(* Logix 5000 AddOnInstructionDefinition export Banner_S15C_UI_Param_v2; software revision 32.00; part 2 of 2 *)
(* tags used below, declared in another part *)
   S15C : Banner_S15C_UI_v2;
   Port_Data : Banner_IOL_Port_v2;
   Port : DINT;
   Local_Control : DINT;
   Command_Being_Processed : BOOL;
   Index_Write_Inprocess : INT;
   Update_Archive : BOOL;
   Inprocess_Index : DINT;
(* Banner_S15C_UI_Param_v2, continued *)

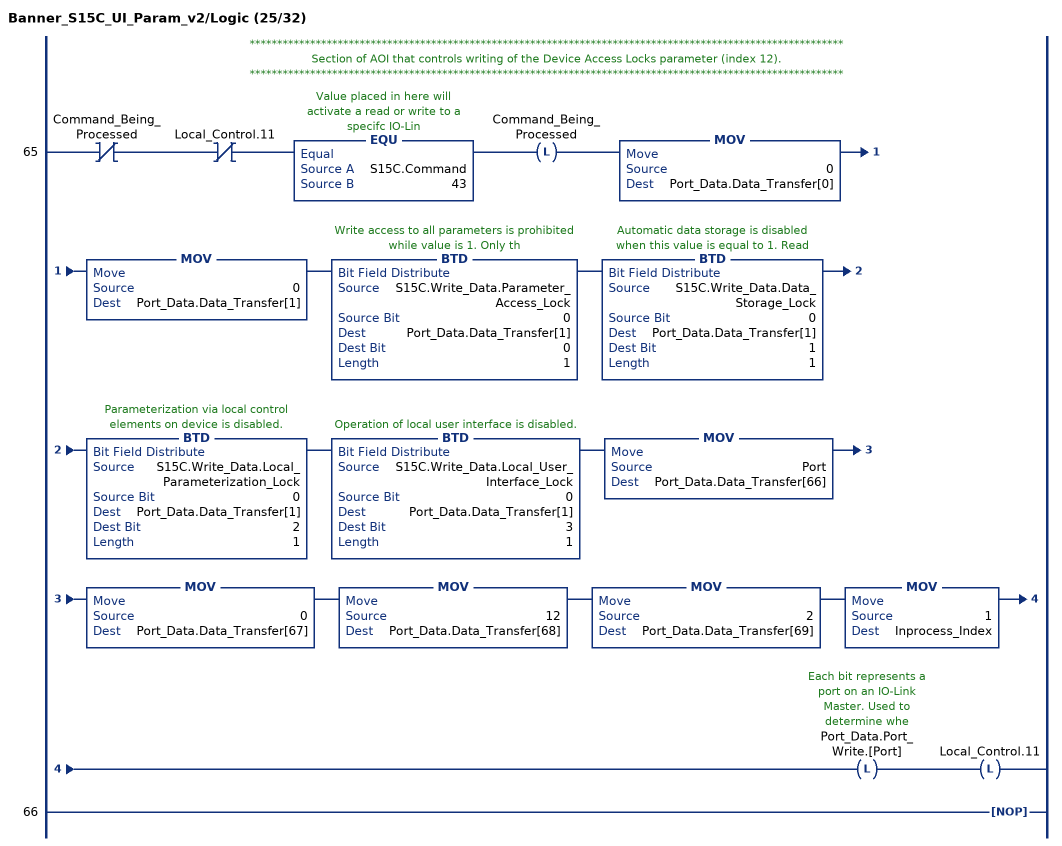
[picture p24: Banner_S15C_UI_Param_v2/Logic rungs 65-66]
   // ************************************************************************************************************
   // Section of AOI that controls writing of the Device Access Locks parameter (index 12).
   // ************************************************************************************************************
   65: XIO(Command_Being_Processed)XIO(Local_Control.11)EQU(S15C.Command,43)OTL(Command_Being_Processed)MOV(0,Port_Data.Data_Transfer[0])MOV(0,Port_Data.Data_Transfer[1])BTD(S15C.Write_Data.Parameter_Access_Lock,0,Port_Data.Data_Transfer[1],0,1)BTD(S15C.Write_Data.Data_Storage_Lock,0,Port_Data.Data_Transfer[1],1,1)BTD(S15C.Write_Data.Local_Parameterization_Lock,0,Port_Data.Data_Transfer[1],2,1)BTD(S15C.Write_Data.Local_User_Interface_Lock,0,Port_Data.Data_Transfer[1],3,1)MOV(Port,Port_Data.Data_Transfer[66])MOV(0,Port_Data.Data_Transfer[67])MOV(12,Port_Data.Data_Transfer[68])MOV(2,Port_Data.Data_Transfer[69])MOV(1,Inprocess_Index)OTL(Port_Data.Port_Write.[Port])OTL(Local_Control.11);
   66: NOP();
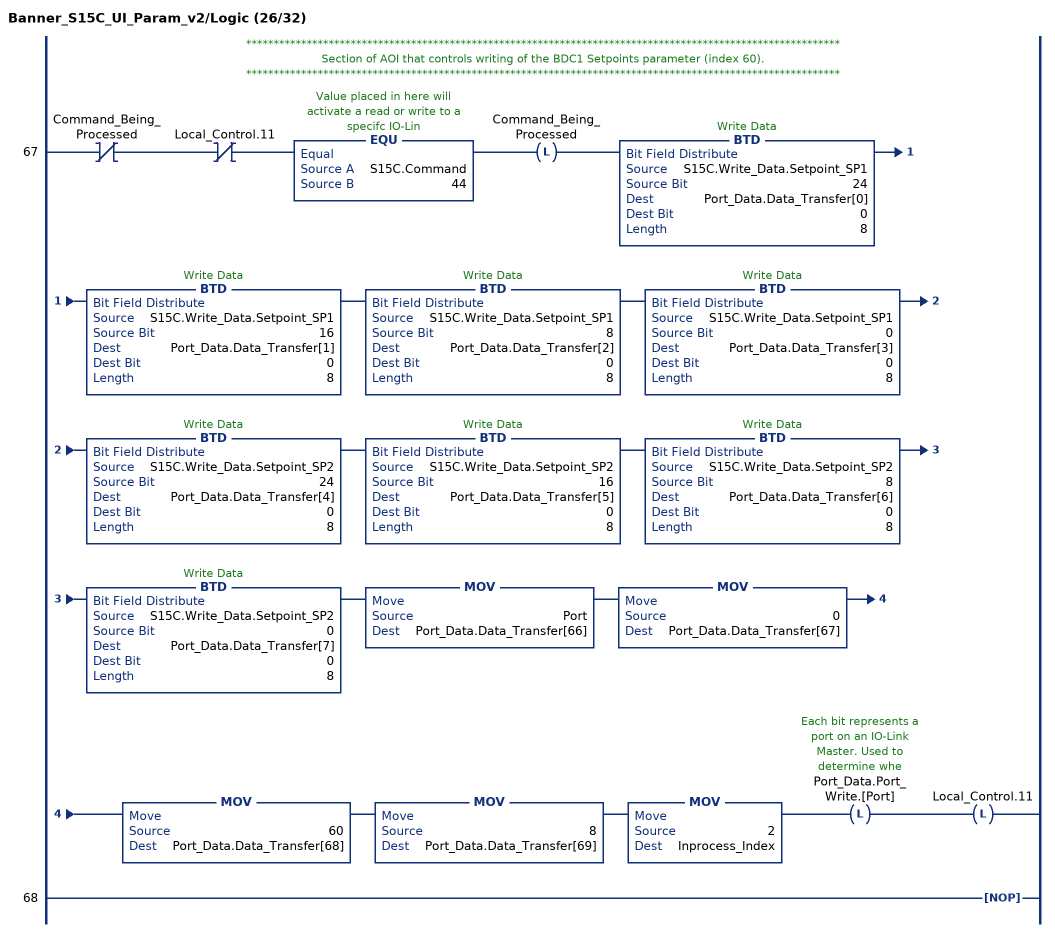
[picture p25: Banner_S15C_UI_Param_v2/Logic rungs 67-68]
   // ************************************************************************************************************
   // Section of AOI that controls writing of the BDC1 Setpoints parameter (index 60).
   // ************************************************************************************************************
   67: XIO(Command_Being_Processed)XIO(Local_Control.11)EQU(S15C.Command,44)OTL(Command_Being_Processed)BTD(S15C.Write_Data.Setpoint_SP1,24,Port_Data.Data_Transfer[0],0,8)BTD(S15C.Write_Data.Setpoint_SP1,16,Port_Data.Data_Transfer[1],0,8)BTD(S15C.Write_Data.Setpoint_SP1,8,Port_Data.Data_Transfer[2],0,8)BTD(S15C.Write_Data.Setpoint_SP1,0,Port_Data.Data_Transfer[3],0,8)BTD(S15C.Write_Data.Setpoint_SP2,24,Port_Data.Data_Transfer[4],0,8)BTD(S15C.Write_Data.Setpoint_SP2,16,Port_Data.Data_Transfer[5],0,8)BTD(S15C.Write_Data.Setpoint_SP2,8,Port_Data.Data_Transfer[6],0,8)BTD(S15C.Write_Data.Setpoint_SP2,0,Port_Data.Data_Transfer[7],0,8)MOV(Port,Port_Data.Data_Transfer[66])MOV(0,Port_Data.Data_Transfer[67])MOV(60,Port_Data.Data_Transfer[68])MOV(8,Port_Data.Data_Transfer[69])MOV(2,Inprocess_Index)OTL(Port_Data.Port_Write.[Port])OTL(Local_Control.11);
   68: NOP();
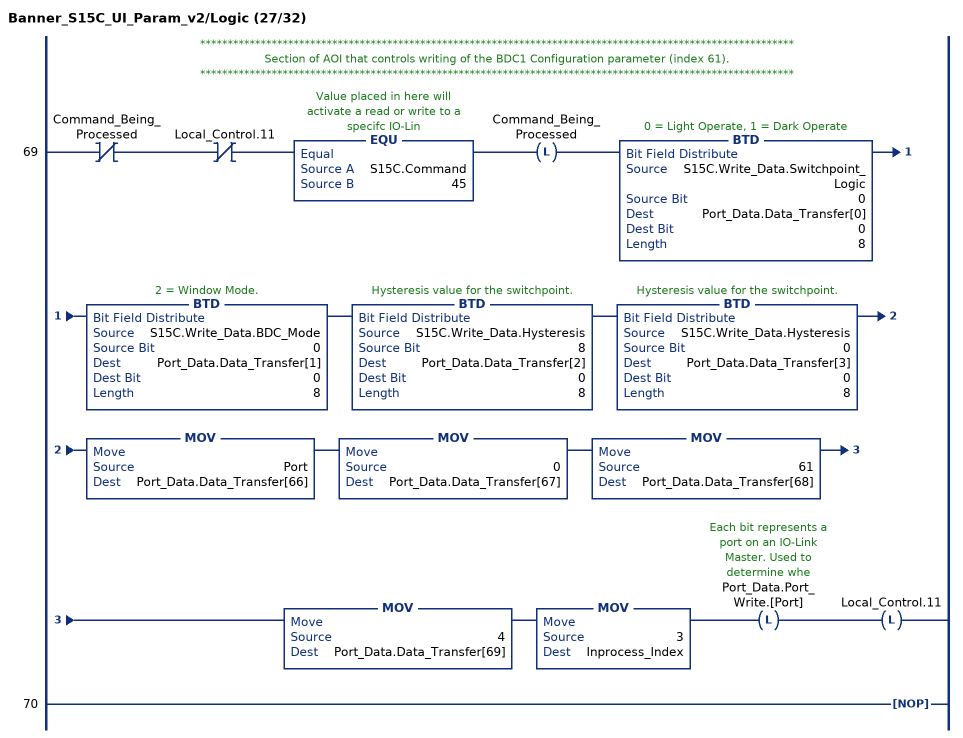
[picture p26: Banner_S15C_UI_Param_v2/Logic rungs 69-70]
   // ************************************************************************************************************
   // Section of AOI that controls writing of the BDC1 Configuration parameter (index 61).
   // ************************************************************************************************************
   69: XIO(Command_Being_Processed)XIO(Local_Control.11)EQU(S15C.Command,45)OTL(Command_Being_Processed)BTD(S15C.Write_Data.Switchpoint_Logic,0,Port_Data.Data_Transfer[0],0,8)BTD(S15C.Write_Data.BDC_Mode,0,Port_Data.Data_Transfer[1],0,8)BTD(S15C.Write_Data.Hysteresis,8,Port_Data.Data_Transfer[2],0,8)BTD(S15C.Write_Data.Hysteresis,0,Port_Data.Data_Transfer[3],0,8)MOV(Port,Port_Data.Data_Transfer[66])MOV(0,Port_Data.Data_Transfer[67])MOV(61,Port_Data.Data_Transfer[68])MOV(4,Port_Data.Data_Transfer[69])MOV(3,Inprocess_Index)OTL(Port_Data.Port_Write.[Port])OTL(Local_Control.11);
   70: NOP();
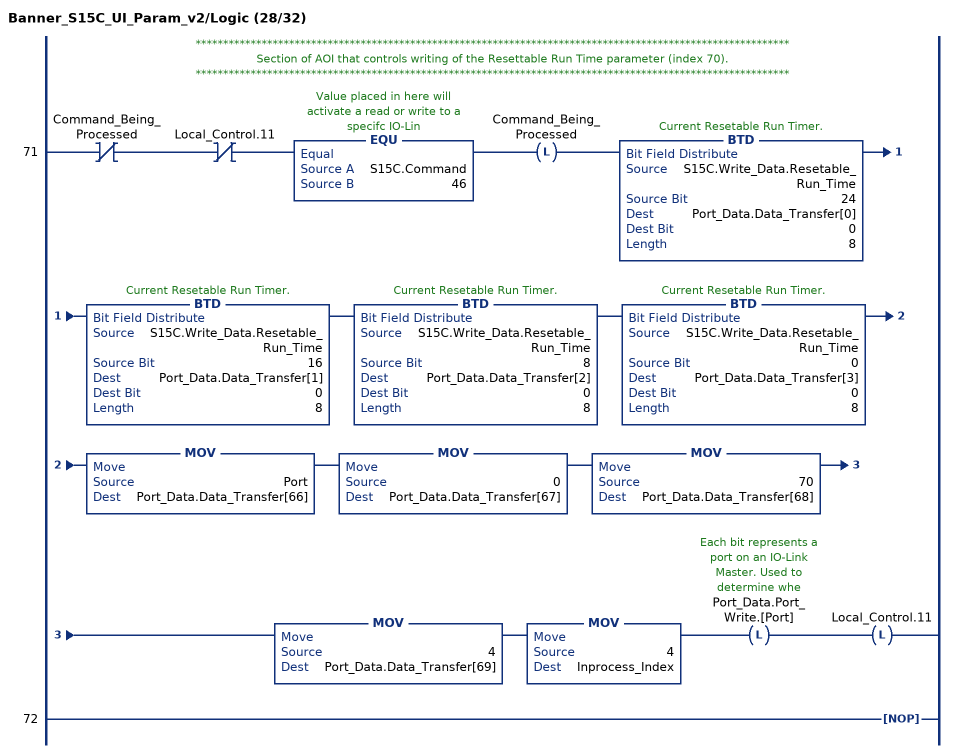
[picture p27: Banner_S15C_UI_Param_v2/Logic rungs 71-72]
   // ************************************************************************************************************
   // Section of AOI that controls writing of the Resettable Run Time parameter (index 70).
   // ************************************************************************************************************
   71: XIO(Command_Being_Processed)XIO(Local_Control.11)EQU(S15C.Command,46)OTL(Command_Being_Processed)BTD(S15C.Write_Data.Resetable_Run_Time,24,Port_Data.Data_Transfer[0],0,8)BTD(S15C.Write_Data.Resetable_Run_Time,16,Port_Data.Data_Transfer[1],0,8)BTD(S15C.Write_Data.Resetable_Run_Time,8,Port_Data.Data_Transfer[2],0,8)BTD(S15C.Write_Data.Resetable_Run_Time,0,Port_Data.Data_Transfer[3],0,8)MOV(Port,Port_Data.Data_Transfer[66])MOV(0,Port_Data.Data_Transfer[67])MOV(70,Port_Data.Data_Transfer[68])MOV(4,Port_Data.Data_Transfer[69])MOV(4,Inprocess_Index)OTL(Port_Data.Port_Write.[Port])OTL(Local_Control.11);
   72: NOP();
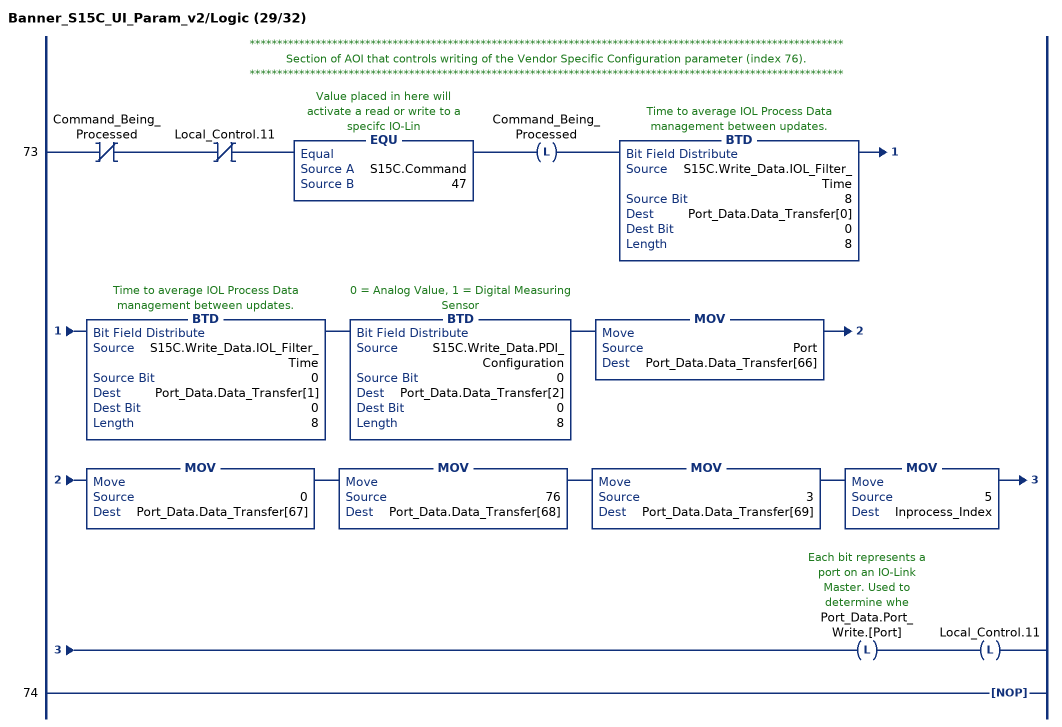
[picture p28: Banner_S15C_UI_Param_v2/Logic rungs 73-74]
   // ************************************************************************************************************
   // Section of AOI that controls writing of the Vendor Specific Configuration parameter (index 76).
   // ************************************************************************************************************
   73: XIO(Command_Being_Processed)XIO(Local_Control.11)EQU(S15C.Command,47)OTL(Command_Being_Processed)BTD(S15C.Write_Data.IOL_Filter_Time,8,Port_Data.Data_Transfer[0],0,8)BTD(S15C.Write_Data.IOL_Filter_Time,0,Port_Data.Data_Transfer[1],0,8)BTD(S15C.Write_Data.PDI_Configuration,0,Port_Data.Data_Transfer[2],0,8)MOV(Port,Port_Data.Data_Transfer[66])MOV(0,Port_Data.Data_Transfer[67])MOV(76,Port_Data.Data_Transfer[68])MOV(3,Port_Data.Data_Transfer[69])MOV(5,Inprocess_Index)OTL(Port_Data.Port_Write.[Port])OTL(Local_Control.11);
   74: NOP();
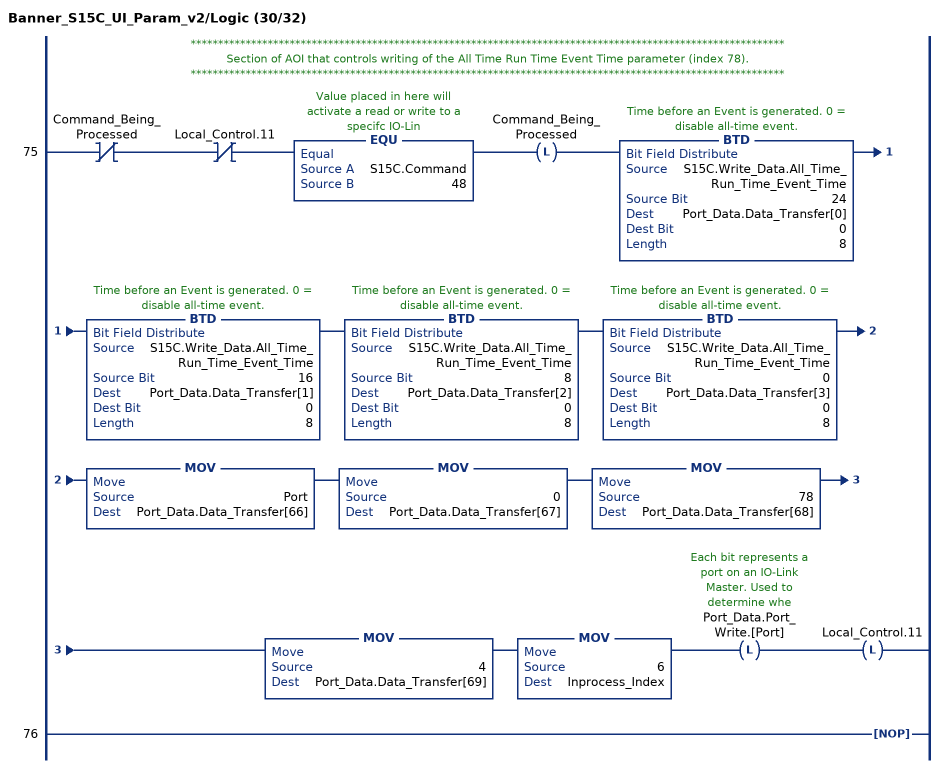
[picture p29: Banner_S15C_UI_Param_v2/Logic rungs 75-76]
   // ************************************************************************************************************
   // Section of AOI that controls writing of the All Time Run Time Event Time parameter (index 78).
   // ************************************************************************************************************
   75: XIO(Command_Being_Processed)XIO(Local_Control.11)EQU(S15C.Command,48)OTL(Command_Being_Processed)BTD(S15C.Write_Data.All_Time_Run_Time_Event_Time,24,Port_Data.Data_Transfer[0],0,8)BTD(S15C.Write_Data.All_Time_Run_Time_Event_Time,16,Port_Data.Data_Transfer[1],0,8)BTD(S15C.Write_Data.All_Time_Run_Time_Event_Time,8,Port_Data.Data_Transfer[2],0,8)BTD(S15C.Write_Data.All_Time_Run_Time_Event_Time,0,Port_Data.Data_Transfer[3],0,8)MOV(Port,Port_Data.Data_Transfer[66])MOV(0,Port_Data.Data_Transfer[67])MOV(78,Port_Data.Data_Transfer[68])MOV(4,Port_Data.Data_Transfer[69])MOV(6,Inprocess_Index)OTL(Port_Data.Port_Write.[Port])OTL(Local_Control.11);
   76: NOP();
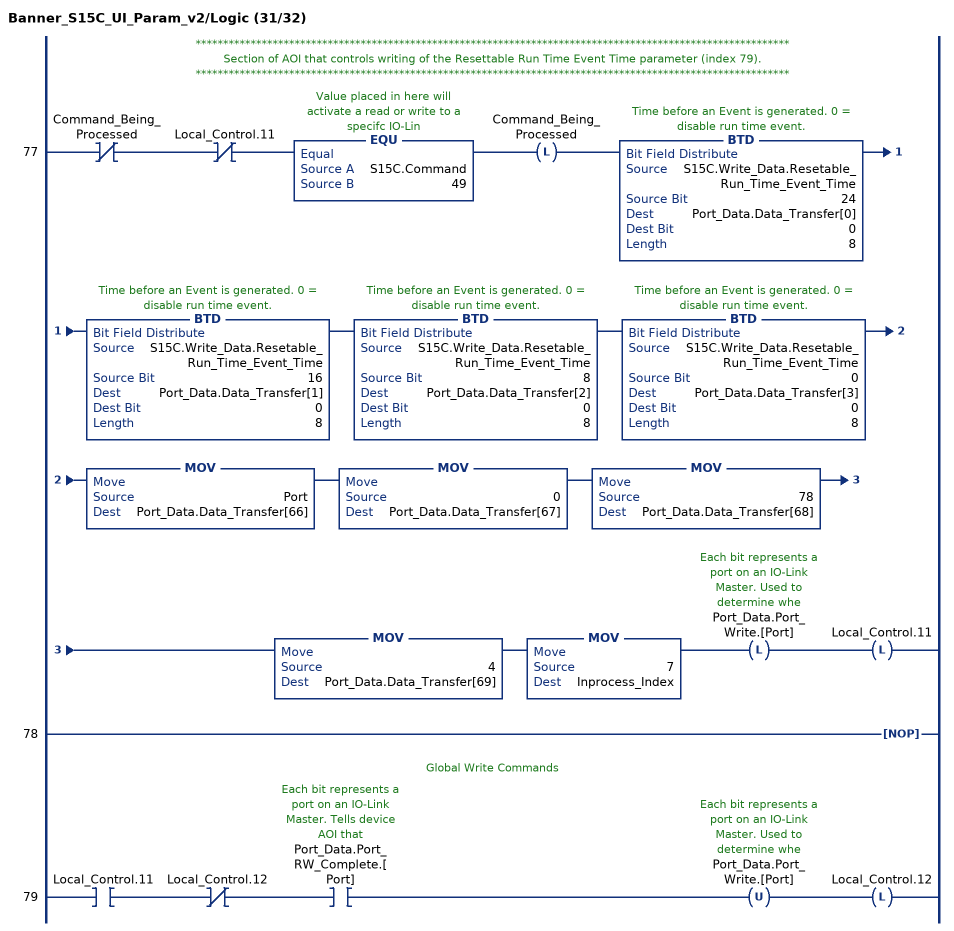
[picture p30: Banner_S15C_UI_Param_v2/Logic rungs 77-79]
   // ************************************************************************************************************
   // Section of AOI that controls writing of the Resettable Run Time Event Time parameter (index 79).
   // ************************************************************************************************************
   77: XIO(Command_Being_Processed)XIO(Local_Control.11)EQU(S15C.Command,49)OTL(Command_Being_Processed)BTD(S15C.Write_Data.Resetable_Run_Time_Event_Time,24,Port_Data.Data_Transfer[0],0,8)BTD(S15C.Write_Data.Resetable_Run_Time_Event_Time,16,Port_Data.Data_Transfer[1],0,8)BTD(S15C.Write_Data.Resetable_Run_Time_Event_Time,8,Port_Data.Data_Transfer[2],0,8)BTD(S15C.Write_Data.Resetable_Run_Time_Event_Time,0,Port_Data.Data_Transfer[3],0,8)MOV(Port,Port_Data.Data_Transfer[66])MOV(0,Port_Data.Data_Transfer[67])MOV(78,Port_Data.Data_Transfer[68])MOV(4,Port_Data.Data_Transfer[69])MOV(7,Inprocess_Index)OTL(Port_Data.Port_Write.[Port])OTL(Local_Control.11);
   78: NOP();
   // Global Write Commands
   79: XIC(Local_Control.11)XIO(Local_Control.12)XIC(Port_Data.Port_RW_Complete.[Port])OTU(Port_Data.Port_Write.[Port])OTL(Local_Control.12);
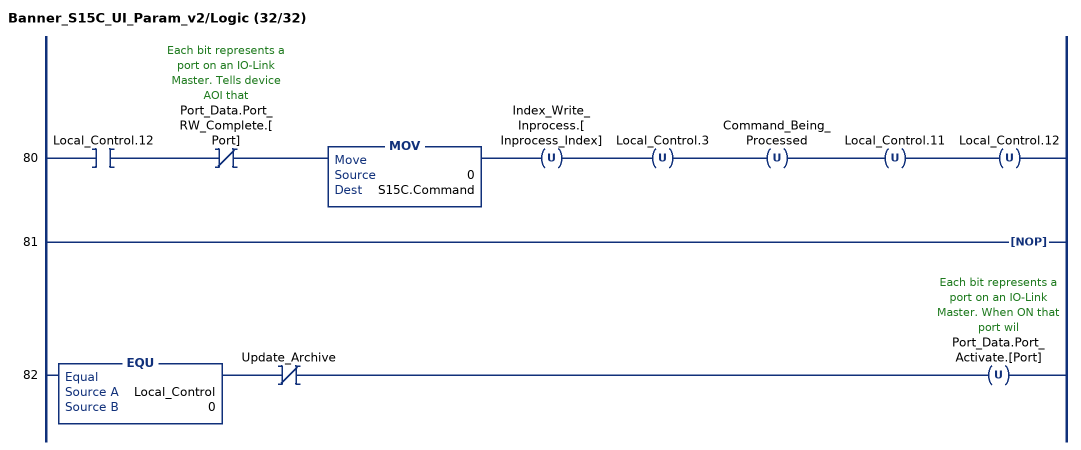
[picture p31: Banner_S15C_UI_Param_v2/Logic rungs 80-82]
   80: XIC(Local_Control.12)XIO(Port_Data.Port_RW_Complete.[Port])MOV(0,S15C.Command)OTU(Index_Write_Inprocess.[Inprocess_Index])OTU(Local_Control.3)OTU(Command_Being_Processed)OTU(Local_Control.11)OTU(Local_Control.12);
   81: NOP();
   82: EQU(Local_Control,0)XIO(Update_Archive)OTU(Port_Data.Port_Activate.[Port]);
END_ROUTINE
END_ADD_ON_INSTRUCTION
